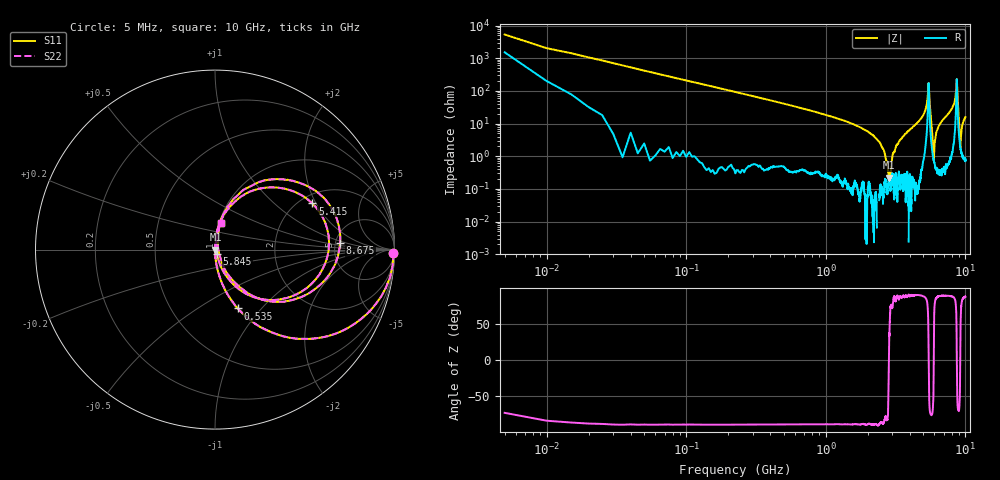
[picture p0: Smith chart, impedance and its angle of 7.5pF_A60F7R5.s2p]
! Amotech Co.,Ltd.
! http://www.amotech.co.kr/
! Part Number: A60F7R5
! These Parameters are Measured in Series Mode Connection
! Operation Temp=25[degC], DC Bias Voltage=0[V]
! Freq. Start=5[MHz] Stop=10[GHz], 2000[Steps]
! Date: Monday, July 20, 2020, 03:31:58
# GHZ S RI R 50.000000
!Freq.(Hz) S11(Real) S11(Imag) S21(Real) S21(Imag) S12(Real) S12(Imag) S22(Real) S22(Imag)
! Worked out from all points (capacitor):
!   2000 points, 5 MHz to 10 GHz, reference 50 ohm
!   read as one part in series: C = 7.64 pF near 55 MHz
!   lowest |Z| = 218 mohm at 2.825 GHz (marker M1)
!   series resonance near 2.834 GHz, so ESL is about 410 pH
!   S11 on the Smith chart (normalised r, x): 5 MHz: open; 535 MHz: 1.01, -0.75; 5.415 GHz: 2.32, +1.87; 5.845 GHz: 1.02, -0.05; 8.675 GHz: 5.51, +0.75; 10 GHz: 1.02, +0.31
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0.005  0.9944 -0.0178  0.00564 0.0178  0.00564 0.0178  0.9944 -0.0178
0.07  0.8974 -0.3011  0.1026 0.3011  0.1026 0.3011  0.8974 -0.3011
0.135  0.7043 -0.4549  0.2957 0.4549  0.2957 0.4549  0.7043 -0.4549
0.535  0.127 -0.3279  0.873 0.3279  0.873 0.3279  0.127 -0.3279
1.675  0.00823 -0.0834  0.9918 0.0834  0.9918 0.0834  0.00823 -0.0834
2.44  0.00172 -0.026  0.9983 0.026  0.9983 0.026  0.00172 -0.026
2.825  0.0021 -0.000568  0.9979 0.000568  0.9979 0.000568  0.0021 -0.000568
3.34  0.00415 0.0274  0.9959 -0.0274  0.9959 -0.0274  0.00415 0.0274
5.005  0.0399 0.1761  0.9601 -0.1761  0.9601 -0.1761  0.0399 0.1761
5.415  0.5421 0.2574  0.4579 -0.2574  0.4579 -0.2574  0.5421 0.2574
5.53  0.3039 -0.2809  0.6961 0.2809  0.6961 0.2809  0.3039 -0.2809
5.845  0.0113 -0.025  0.9887 0.025  0.9887 0.025  0.0113 -0.025
5.94  0.00716 0.0014  0.9928 -0.0014  0.9928 -0.0014  0.00716 0.0014
6.185  0.00699 0.0518  0.993 -0.0518  0.993 -0.0518  0.00699 0.0518
6.67  0.0149 0.1061  0.9851 -0.1061  0.9851 -0.1061  0.0149 0.1061
8.335  0.1824 0.3449  0.8176 -0.3449  0.8176 -0.3449  0.1824 0.3449
8.555  0.4593 0.3755  0.5407 -0.3755  0.5407 -0.3755  0.4593 0.3755
8.675  0.6967 0.035  0.3033 -0.035  0.3033 -0.035  0.6967 0.035
8.8  0.3304 -0.2898  0.6696 0.2898  0.6696 0.2898  0.3304 -0.2898
9.19  0.0182 0.00205  0.9818 -0.00205  0.9818 -0.00205  0.0182 0.00205
9.49  0.018 0.0825  0.982 -0.0825  0.982 -0.0825  0.018 0.0825
10  0.0315 0.1508  0.9685 -0.1508  0.9685 -0.1508  0.0315 0.1508
